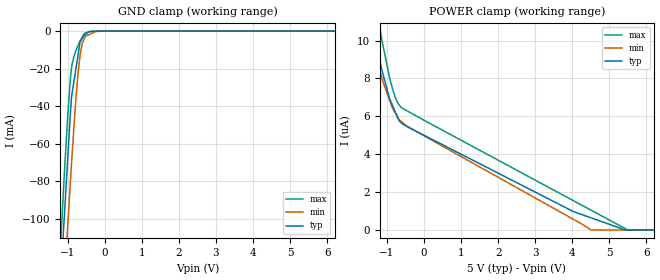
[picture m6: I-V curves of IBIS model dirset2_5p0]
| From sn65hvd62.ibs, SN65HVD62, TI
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|   dirset2_5p0 Model
[Model]   dirset2_5p0
Model_type   Input
Vinl = 1.5
Vinh = 3.5
|   typ   min   max
|   (nom PVT)   (fast PVT)   (slow PVT)
 C_comp   1.340e-12   1.316e-12   1.391e-12
| Where nom  PVT is Nominal Process, 5V, 27C
|   Fast PVT is Strong Process,  5.5V, -40C
|   Slow PVT is Weak Process,   4.5V, 125C
[Voltage Range]   5   4.5   5.5
|Ambient Temperature   25   85   -40
|Junction Temperature
[Temperature Range]   27   125   -40
[Power Clamp Reference]   5   4.5   5.5
[GND Clamp Reference]   0   0   0
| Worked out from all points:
|   GND clamp passes 1 mA (typ) near -0.48 V on its own axis
[GND Clamp]
|   Voltage   I(typ)   I(min)   I(max)
-5V       -1.666A    -1.639A    -1.693A
-1.183V   -129.6mA   -165mA     -108.6mA
-1.14V    -113.6mA   -149.9mA   -92.65mA
-1.089V   -96.51mA   -132.3mA   -73.94mA
-1.022V   -73.91mA   -109.4mA   -51.19mA
-935mV    -44.94mA   -81.43mA   -26.12mA
-885.5mV  -33.06mA   -65.82mA   -17.66mA
-792mV    -21.26mA   -38.53mA   -10.88mA
-670.5mV  -5.924mA   -12.78mA   -5.244mA
-607.5mV  -3.895mA   -6.372mA   -3.091mA
-435mV    -300.5uA   -1.947mA   -463.2uA
10V       0A         0A         0A
[POWER Clamp]
|   Voltage   I(typ)   I(min)   I(max)
-5V       28.08uA    20.77uA    39.66uA
-1.521V   12.13uA    10.72uA    14.7uA
-1.373V   10.56uA    9.672uA    12.76uA
-1.14V    8.453uA    8.03uA     10.04uA
-935mV    6.942uA    6.872uA    8.075uA
-841.5mV  6.524uA    6.391uA    7.375uA
-693mV    5.86uA     5.872uA    6.64uA
-605mV    5.633uA    5.71uA     6.447uA
4.02V     979.7nA    572.7nA    1.557uA
4.505V    643.1nA    0A         1.047uA
5.495V    0A         0A         0A
10V       0A         0A         0A
